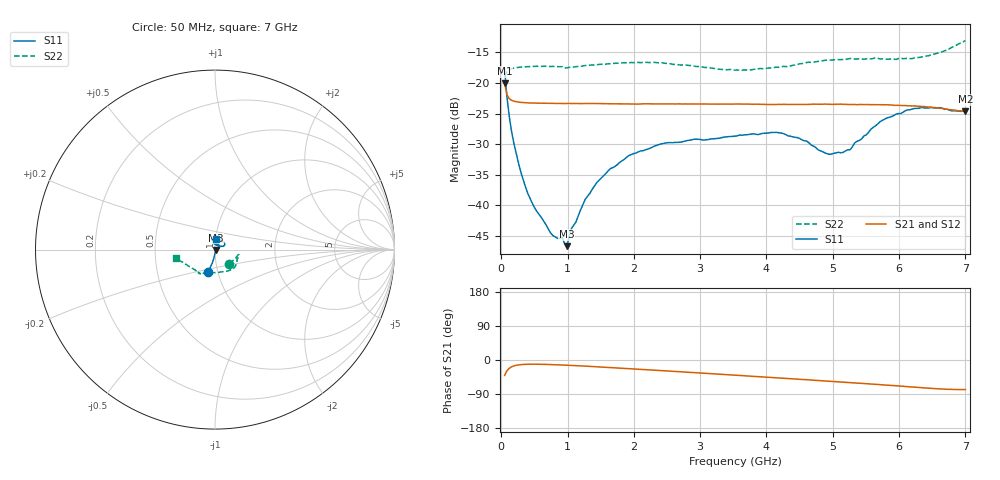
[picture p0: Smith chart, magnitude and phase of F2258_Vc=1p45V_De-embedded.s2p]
! Integrated Device Technology
! Corporate Headquarters
! 6024 Silver Creek Valley Road
! San Jose, CA 95138  USA
! Phone:  1-408-284-8200
! Toll Free:  1-800-223-1366
! Webpage:  http://www.idt.com/
! Timing and RF Division
! 515 Groton Road, Suite 102
! Westford, MA 01886-6024
! Device:  F2258
! Description: Voltage Variable RF Attenuator
! Frequency:  50.0 -  6000.00 MHz
! Package:  3x3 mm Thin QFN Plastic Package: 16 pin
! Ports:  2 RF, 2 DC
!  Pin  1  = NC
!  Pin  2  = NC
!  Pin  3  = RF2  = Port 2
!  Pin  4  = GND
!  Pin  5  = Vdd
!  Pin  6  = NC
!  Pin  7  = VCTRL
!  Pin  8  = NC
!  Pin  9  = GND
!  Pin 10  = RF1  = Port 1
!  Pin 11  = NC
!  Pin 12  = NC
!  Pin 13  = NC
!  Pin 14  = NC
!  Pin 15  = NC
!  Pin 16  = NC
! Vcntrl:  1.450 Volts
! Vdd:  +3.300 Volts
! Current:  1.161 mA
! Data:  The device was measured on a the F2258 evaluation board which has
!  individual transmission lines to the RF pins.  Data was collected
!  using a calibrated network analyzer.  The evaluation board was
!  de-embedded using a TRL calibration technique.
!  The reference plane is the edge of the package pin.
! Misc:  SN 10
!  Action Tracker AT0285
! Date Measured:  2014-12-10
! Date:  2016-01-13  MJV
! Note:
!  Integrated Device Technology supplies this data as a sample of measured
!  data at the package pin for this product.  Your particular data for this
!  product may vary.
!  Data was taken at 25 degrees C.
!  Integrated Device Technology reserves the right to change this data at anytime.
!Freq_(GHz)  S11M_(dB)  S11P_(deg)  S21M_(dB)  S21P_(deg)  S12M_(dB)  S12P_(deg)  S22M_(dB)  S22P_(deg)
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# GHz S dB R 50
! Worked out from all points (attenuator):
!   201 points, 50 MHz to 7 GHz, reference 50 ohm
!   highest |S21| = -20.06 dB at 50 MHz (marker M1); lowest = -24.6 dB at 7 GHz (marker M2)
!   lowest |S11| = -46.7 dB at 988.2 MHz (marker M3), VSWR 1.01, Z = 50.4 - j0.262 ohm
!   |S11| at or under -10 dB: start of sweep to end of sweep
!   |S22| runs from -18.9 to -13.0 dB; largest |S21 - S12| = 0.00048
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0.05  -17.73 -107.2  -20.06 -40.6  -20.06 -40.6  -18.95 -44.5
0.08475  -22.22 -101.6  -21.91 -28.5  -21.91 -28.5  -18.17 -23.0
0.15425  -27.89 -97.0  -22.83 -18.1  -22.81 -18.1  -17.65 -14.1
0.2585  -33.08 -92.0  -23.12 -13.0  -23.11 -13.0  -17.44 -11.6
0.3975  -38.02 -84.5  -23.25 -11.2  -23.23 -11.2  -17.32 -12.2
0.745  -44.55 -46.3  -23.34 -12.0  -23.33 -12.0  -17.30 -18.0
0.91875  -45.25 -8.1  -23.35 -13.2  -23.36 -13.2  -17.32 -22.0
0.98825  -46.70 -34.3  -23.35 -13.7  -23.34 -13.7  -17.52 -23.2
1.05775  -43.81 -15.7  -23.36 -14.3  -23.34 -14.3  -17.42 -24.5
1.2315  -39.87 2.1  -23.36 -15.8  -23.34 -15.8  -17.20 -27.8
1.44  -36.30 8.2  -23.36 -18.0  -23.38 -18.0  -17.01 -31.6
1.6485  -33.99 13.4  -23.40 -20.1  -23.37 -20.1  -16.85 -35.3
1.9265  -31.86 22.5  -23.43 -22.9  -23.43 -22.9  -16.67 -40.2
2.37825  -30.07 34.2  -23.43 -27.6  -23.45 -27.6  -16.68 -48.5
3.525  -28.70 84.8  -23.45 -40.1  -23.45 -40.1  -17.89 -82.7
4.1505  -28.08 102.5  -23.51 -47.0  -23.46 -47.1  -17.40 -105.3
4.7065  -30.32 92.4  -23.46 -53.3  -23.46 -53.3  -16.59 -117.0
4.94975  -31.67 73.6  -23.50 -56.0  -23.51 -56.0  -16.26 -119.4
5.15825  -31.34 53.4  -23.49 -58.6  -23.51 -58.5  -16.14 -121.1
5.85325  -25.62 23.1  -23.58 -66.9  -23.58 -66.9  -16.09 -127.9
6.33975  -23.98 30.1  -23.85 -73.2  -23.83 -73.2  -15.76 -140.1
7  -24.32 83.6  -24.64 -77.9  -24.61 -78.0  -13.03 -168.1
